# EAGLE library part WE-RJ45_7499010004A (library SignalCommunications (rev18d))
Order Code 7499010004A Design THT xBase-T 10/100 Base-T Ports 1x1 Application Standard Tab Position Down LED (Left-Right) NONE EMI Fingers No Details see: http://katalog.we-online.de/en/pbs/WE-LAN_RJ45/7499010004A? Updated by Yingchun Shan 2016-08-26 2016(C) Würth Elektronik
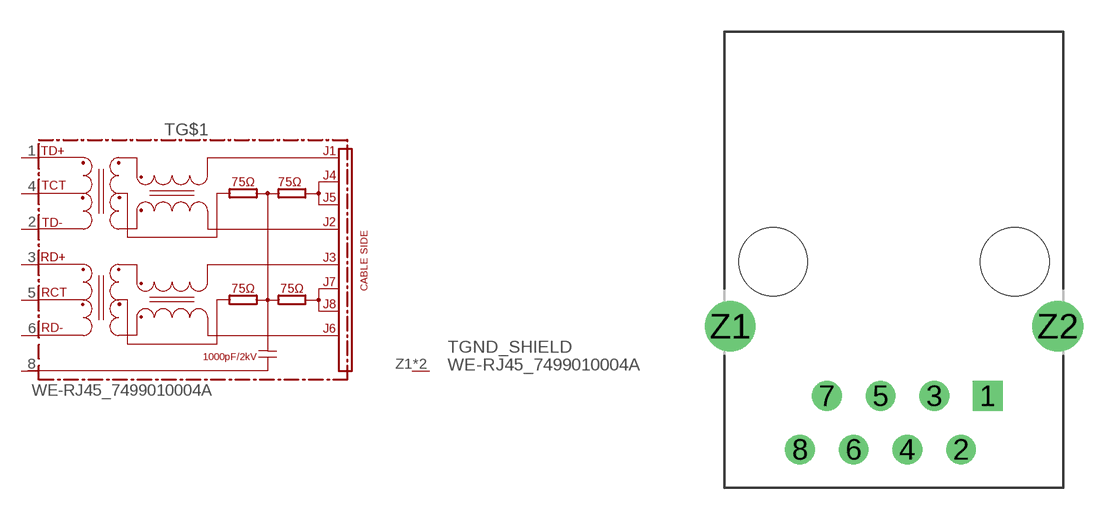
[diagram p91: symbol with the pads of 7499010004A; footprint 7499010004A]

Designator prefix T; gates GND_SHIELD=GNDPIN G$1=74990X-THT-10/100-T

## WE-RJ45_7499010004A (COMPANY-URL: http://www.we-online.de; CREATED-BY: Christin Zierenner; CREATED-DATE: AUG 2012; DATASHEET-URL: http://katalog.we-online.de/kataloge/eisos/media/pdf/7499010004A.pdf; MANUFACTURER: Würth Elektronik eiSos GmbH)  [7499010004A]
1  G$1:TD+
2  G$1:TD-
3  G$1:RD+
4  G$1:TCT
5  G$1:RCT
6  G$1:RD-
8  G$1:8
Z1  GND_SHIELD:GND  pwr
Z2  GND_SHIELD:GND  pwr

## Footprint 7499010004A (pad centres in mm)
MAX HEIGHT=13.74mm PORTS----1X1 LED --NO
drill 0.9 square: 1 4.445,-6.35
drill 0.9: 2 3.175,-8.89; 3 1.905,-6.35; 4 0.635,-8.89; 5 -0.635,-6.35; 6 -1.905,-8.89; 7 -3.175,-6.35; 8 -4.445,-8.89
drill 1.6: Z1 -7.745,-3.05; Z2 7.745,-3.05
hole 3.25 at 5.715,0
hole 3.25 at -5.715,0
